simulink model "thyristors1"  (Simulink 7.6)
settings: Solver=ode23s  StartTime=0.0  StopTime=0.04  RelTol=1e-3
InitFcn:
  | Couple=0;
  | ton=0.5;
  | toff=3;
StopFcn:
  | close all
  | load Ug_et_Us.mat
  | subplot 211
  | plot(x(1,:),x(2,:))
  | grid
  | axis([0 0.04 -0.2 1.2])
  | title('commande gâchette')
  | xlabel('temps')
  | 
  | subplot 212
  | plot(x(1,:),x(3,:),x(1,:),x(4,:))
  | title('tension aux bornes de la charge R et sinusoïde d''entrée')
  | grid
  | xlabel('temps')
  | 
  | % =============================================
  | figure(2)
  | load Iak_et_Vak.mat
  | 
  | subplot 211
  | plot(y(1,:),y(2,:))
  | grid
  | %axis([0 0.04 -0.2 1.2])
  | title('courant Iak et tension Vak')
  | xlabel('temps')
  | 
  | subplot 212
  | plot(y(1,:),y(3,:))
  | grid
  | title('courant Iak et tension Vak')
  | xlabel('temps')
  | 
  | % =============================================
  | figure(3)
  | load Us_et_MoyUs.mat
  | plot(z(1,:),z(2,:),z(1,:),z(3,:))
  | grid
  | title('tension de sortie et sa valeur moyenne')
  | xlabel('temps')
libraries: powerlib x7, powerlib_extras x1

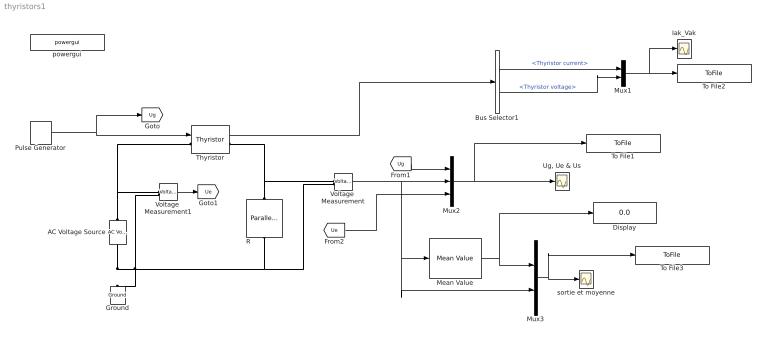
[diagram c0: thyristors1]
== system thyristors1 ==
  AC Voltage Source : powerlib/Electrical Sources/AC Voltage Source  DialogController=POWERSYS.PowerSysDialog  SystemSampleTime=-1  Amplitude=100  Phase=0  Frequency=60  SampleTime=0  Measurements=None
  Bus Selector1 : BusSelector  OutputSignals=Thyristor current,Thyristor voltage
  Display : Display
  Ground : powerlib/Elements/Ground  DialogController=POWERSYS.PowerSysDialog  PhysicalDomain=powersysdomain  SubClassName=unknown  LeftPortType=p1  RightPortType=p1  LConnTagsString=a
  Iak_Vak : Scope
  Mean Value : powerlib_extras/Measurements/Mean Value  DialogController=POWERSYS.PowerSysDialog  SystemSampleTime=-1  Period=1/60
  Mux1 : Mux  Inputs=2
  Mux2 : Mux  Inputs=3
  Mux3 : Mux  Inputs=2
  Pulse Generator : DiscretePulseGenerator  PulseType=Time based  Period=(1-0.2)/60/3  PulseWidth=2
  R : powerlib/Elements/Parallel RLC Branch  DialogController=POWERSYS.PowerSysDialog  PhysicalDomain=powersysdomain  SubClassName=unknown  LeftPortType=p1  RightPortType=p1  LConnTagsString=a  RConnTagsString=__new0  BranchType=R  Resistance=10  Inductance=1e-3  SetiL0=off  InitialCurrent=0  Capacitance=1e-6  Setx0=off  InitialVoltage=0  Measurements=None
  Thyristor : powerlib/Power Electronics/Thyristor  DialogController=POWERSYS.PowerSysDialog  SystemSampleTime=-1  Ron=0.001  Lon=0  Vf=0.8  IC=0  Rs=500  Cs=250e-9  Measurements=on
  To File1 : ToFile  Filename=Ug_et_Us  MatrixName=x
  To File2 : ToFile  Filename=Iak_et_Vak  MatrixName=y
  To File3 : ToFile  Filename=Us_et_MoyUs  MatrixName=z
  "Ug, Ue & Us" : Scope
  Voltage  Measurement : powerlib/Measurements/Voltage Measurement  DialogController=POWERSYS.PowerSysDialog  SystemSampleTime=-1  PhasorSimulation=off  OutputType=Complex  PSBequivalent=0
  Voltage  Measurement1 : powerlib/Measurements/Voltage Measurement  DialogController=POWERSYS.PowerSysDialog  SystemSampleTime=-1  PhasorSimulation=off  OutputType=Complex  PSBequivalent=0
  powergui : powerlib/powergui  Priority=1  SystemSampleTime=-1  SimulationMode=Continuous  SampleTime=50e-6  frequency=60  SPID=off  DisableSnubberDevices=off  DisableRonSwitches=off  DisableVfSwitches=off  SwTol=0  Interpol=off  frequencyindice=0  echomessages=off  HookPort=off  DisplayEquations=off  FunctionMessages=off  EnableUseOfTLC=off  x0status=blocks  RestoreLinks=warning  ResistiveCurrentMeasurement=off  Ylog=off  Xlog=on  ShowGrid=off  save=off  variable=ZData  ZoomFFT=off  StartTime=0.0  cycles=1  DisplayStyle=1  fundamental=60  FreqAxis=off  MaxFrequency=1000  frequencyindicesteady=1  display=off  methode=off
  sortie et moyenne : Scope
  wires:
  Pulse Generator/1 -> Thyristor/1, [Ug]
  Thyristor/1 -> Bus Selector1/1
  Bus Selector1/1 -> Mux1/1  "<Thyristor current>"
  Bus Selector1/2 -> Mux1/2  "<Thyristor voltage>"
  Mux1/1 -> To File2/1, Iak_Vak/1
  Voltage  Measurement/1 -> Mux2/2, Mean Value/1, Mux3/2
  Mux2/1 -> "Ug, Ue & Us"/1, To File1/1
  [Ug] -> Mux2/1
  Voltage  Measurement1/1 -> [Ue]
  [Ue] -> Mux2/3
  Mean Value/1 -> Mux3/1, Display/1
  Mux3/1 -> sortie et moyenne/1, To File3/1
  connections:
  AC Voltage Source/RConn1 -- Thyristor/LConn1 -- Voltage  Measurement1/LConn1
  AC Voltage Source/LConn1 -- Ground/LConn1 -- R/LConn1 -- Voltage  Measurement/LConn2 -- Voltage  Measurement1/LConn2
  R/RConn1 -- Thyristor/RConn1 -- Voltage  Measurement/LConn1
